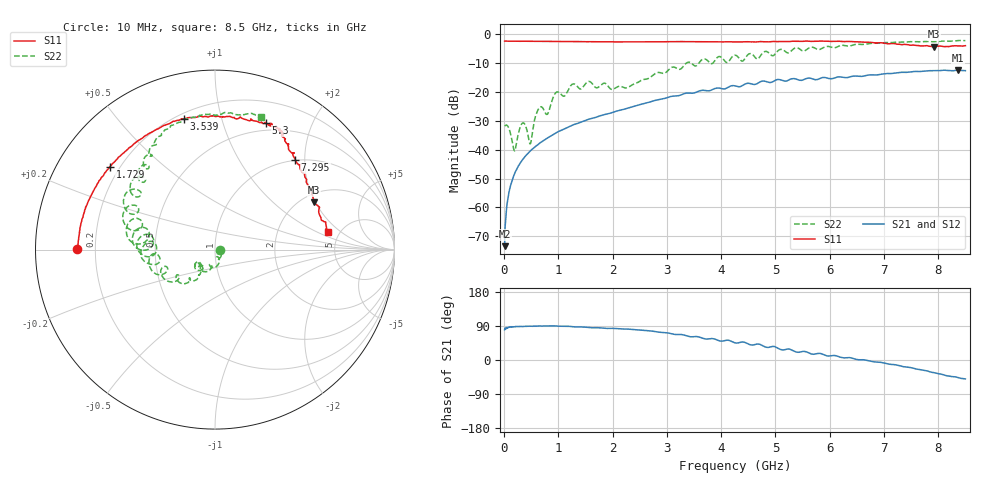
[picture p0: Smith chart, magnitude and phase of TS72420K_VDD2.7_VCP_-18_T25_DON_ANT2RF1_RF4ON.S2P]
!Agilent Technologies,E5071C,MY46417908,A.11.23
!Date: Thu Oct 03 16:41:38 2019
!Data & Calibration Information:
!Freq	S11:SOLT2(ON)	S21:SOLT2(ON)	S12:SOLT2(ON)	S22:SOLT2(ON)
!PortZ  Port1:50+j0  Port2:50+j0
!Above PortZ is port z conversion or system Z0 setting when saving the data.
!When reading, reference impedance value at option line is always used.
# Hz S dB R 50
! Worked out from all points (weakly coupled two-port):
!   1601 points, 10 MHz to 8.5 GHz, reference 50 ohm
!   highest |S21| = -12.36 dB at 8.357 GHz (marker M1); lowest = -73.5 dB at 10 MHz (marker M2)
!   lowest |S11| = -4.3 dB at 7.922 GHz (marker M3), VSWR 4.16, Z = 116 + j97.8 ohm
!   |S11| at or under -10 dB: nowhere
!   |S22| runs from -40.4 to -2.1 dB; largest |S21 - S12| = 0.0032
!   S11 on the Smith chart (normalised r, x): 10 MHz: 0.13, +0.00; 1.729 GHz: 0.16, +0.34; 3.539 GHz: 0.23, +0.77; 5.3 GHz: 0.42, +1.39; 7.295 GHz: 0.99, +1.80; 8.5 GHz: 4.04, +1.36
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1e7  -2.31 179.9  -73.47 79.8  -73.02 75.8  -31.75 -2.0
1.108188e8  -2.34 177.5  -53.04 86.4  -53.18 86.9  -33.83 -38.9
1.957188e8  -2.36 175.5  -48.22 87.8  -48.32 87.4  -40.41 -20.2
3.230688e8  -2.37 172.5  -43.91 88.6  -43.97 88.6  -31.11 -29.8
4.822562e8  -2.38 169.1  -40.46 89.0  -40.51 89.0  -37.94 -41.7
6.520562e8  -2.40 165.3  -37.81 89.7  -37.84 89.7  -25.41 -57.2
7.900188e8  -2.42 162.4  -36.06 89.8  -36.09 89.6  -27.77 -74.4
9.598188e8  -2.43 158.7  -34.10 89.7  -34.14 89.5  -20.10 -90.7
1.426769e9  -2.51 148.4  -30.36 87.1  -30.37 86.9  -18.80 -126.0
1.559425e9  -2.52 145.3  -29.43 85.5  -29.42 85.4  -16.32 -133.7
1.729225e9  -2.54 141.7  -28.50 85.2  -28.47 85.1  -18.41 -136.1
2.25985e9  -2.60 129.6  -25.68 81.5  -25.63 81.5  -18.53 -127.5
2.843538e9  -2.57 116.6  -22.66 73.6  -22.61 73.7  -13.19 -129.1
3.538656e9  -2.51 103.2  -20.07 62.0  -20.06 62.2  -10.90 -157.7
4.255e9  -2.58 88.4  -17.86 45.4  -17.85 45.5  -7.21 176.2
5.300331e9  -2.38 68.2  -15.39 26.3  -15.37 26.4  -5.57 156.8
5.671769e9  -2.41 64.0  -15.36 15.6  -15.35 15.8  -4.43 139.2
7.088538e9  -3.25 51.6  -13.57 -10.9  -13.60 -10.9  -2.83 111.6
7.295481e9  -3.47 48.2  -13.19 -15.4  -13.23 -15.8  -2.68 107.0
7.921619e9  -4.26 25.6  -12.60 -33.4  -12.49 -33.4  -2.51 89.6
8.356731e9  -3.98 12.2  -12.36 -46.1  -12.42 -46.1  -2.14 75.9
8.5e9  -3.91 9.0  -12.57 -49.9  -12.64 -49.8  -2.14 70.9
